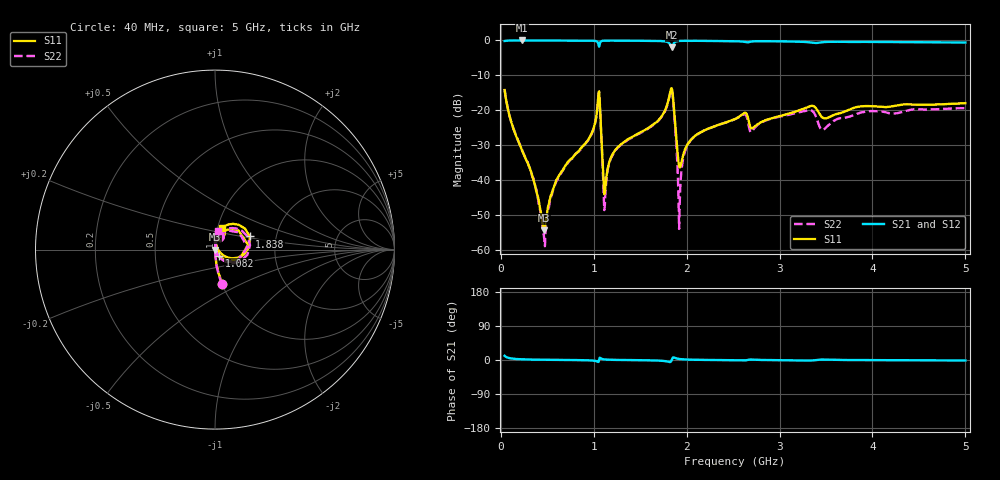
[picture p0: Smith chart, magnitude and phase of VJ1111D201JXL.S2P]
! VJ1111D201JXL
! DATE 02/15/2022  13:22
! CAPACITORS MOUNTED IN SERIES ON 25 MIL THICK MICROSTRIP SUBSTRATE
# GHz  S  MA  R  50.00
!  FREQ  S11M  S11A  S21M  S21A  S12M  S12A  S22M  S22A
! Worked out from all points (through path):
!   801 points, 40 MHz to 5 GHz, reference 50 ohm
!   highest |S21| = -0.01 dB at 226 MHz (marker M1); lowest = -2.0 dB at 1.838 GHz (marker M2)
!   lowest |S11| = -54.4 dB at 467.8 MHz (marker M3), VSWR 1.00, Z = 50.2 + j0.0326 ohm
!   |S11| at or under -10 dB: start of sweep to end of sweep
!   |S22| runs from -59.0 to -14.0 dB; largest |S21 - S12| = 0.01
!   S11 on the Smith chart (normalised r, x): 40 MHz: 1.01, -0.40; 1.082 GHz: 1.05, -0.07; 1.838 GHz: 1.46, +0.22; 5 GHz: 1.06, +0.26
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0.04  0.1948 -77.8  0.9804 11.2  0.9806 11.4  0.1986 -77.9
0.226  0.02694 -84.5  0.9984 1.9  0.9979 1.8  0.0276 -86.1
0.3624  0.008683 -75.0  0.9953 1.0  1 1.0  0.009199 -79.0
0.4678  0.001897 9.9  0.9965 0.6  0.9994 0.8  0.001383 3.4
0.598  0.01009 77.4  0.9949 0.3  0.9995 0.2  0.009555 79.0
0.8708  0.02909 83.9  0.9931 -0.4  0.9966 -0.3  0.02882 84.3
1.0444  0.1334 57.1  0.9262 -5.1  0.9283 -5.1  0.1303 54.0
1.0816  0.04117 -54.7  0.9764 3.6  0.9795 3.6  0.03922 -61.2
1.1002  0.0126 -43.2  0.9892 2.1  0.9919 2.1  0.01077 -56.1
1.125  0.00785 52.4  0.9921 1.3  0.9943 1.3  0.00658 67.1
1.2428  0.02797 84.4  0.9921 0.3  0.9968 0.2  0.02746 85.5
1.6954  0.07185 84.0  0.9821 -1.6  0.9867 -1.7  0.07062 79.4
1.838  0.2071 20.8  0.7959 -0.2  0.7997 -0.2  0.1968 7.3
1.9248  0.01509 24.1  0.9839 2.6  0.9885 2.5  0.004471 77.8
1.9744  0.02571 73.4  0.9866 1.5  0.9918 1.5  0.02384 92.1
2.0488  0.0382 82.3  0.9855 0.9  0.9932 0.8  0.03797 90.6
2.52  0.07486 82.7  0.9752 -0.7  0.9807 -0.8  0.07461 84.1
2.6998  0.05482 67.7  0.9647 1.1  0.9703 1.0  0.04914 75.1
3.3508  0.1157 68.4  0.9286 -1.2  0.9335 -1.4  0.09772 63.1
3.4624  0.07835 63.2  0.9416 1.1  0.9467 0.9  0.05223 71.7
4.1754  0.1117 74.3  0.9475 -0.6  0.9536 -0.7  0.09078 82.5
5  0.1262 70.8  0.9321 -1.2  0.9367 -1.5  0.1071 80.0
